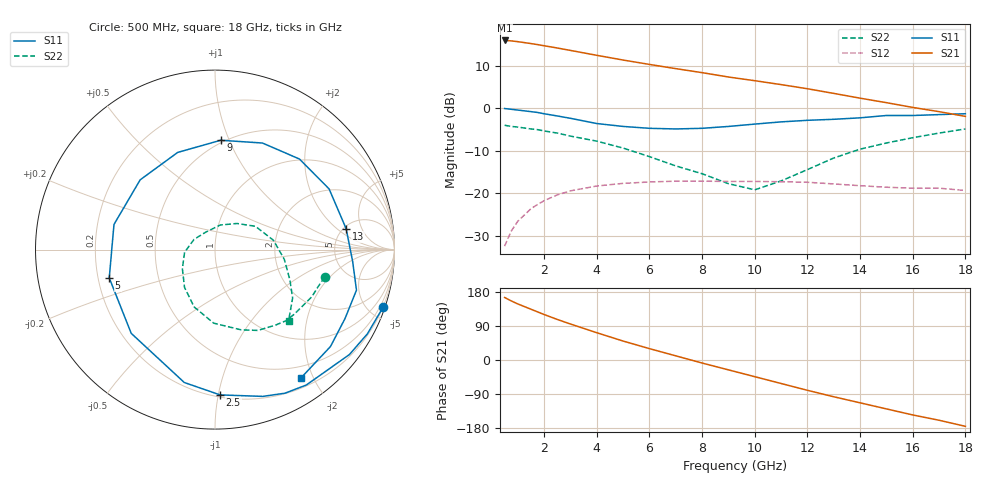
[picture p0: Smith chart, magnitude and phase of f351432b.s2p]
!ATF-35143
!S-PARAMETERS at Vds=2V  Id=10mA.  LAST UPDATED 06-3-99
# ghz s ma r 50
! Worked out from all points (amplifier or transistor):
!   23 points, 500 MHz to 18 GHz, reference 50 ohm
!   highest |S21| = 15.9 dB at 500 MHz (marker M1)
!   |S21| within 3 dB of that: start of sweep to 3.576 GHz
!   unconditionally stable (mu >= 1): 8.306 GHz to end of sweep
!   at 1.5 GHz: K = 0.23, MSG = 19.4 dB, |S12| = -23.6 dB
!   at 7 GHz: K = 0.88, MSG = 13.2 dB, |S12| = -17.1 dB
!   at 18 GHz: K = 1.41, MAG = 4.9 dB, |S12| = -19.3 dB
!   lowest NFmin = 0.10 dB at 500 MHz
!   S11 on the Smith chart (normalised r, x): 500 MHz: 0.18, -5.97; 2.5 GHz: 0.21, -1.01; 5 GHz: 0.25, -0.12; 9 GHz: 0.48, +0.93; 13 GHz: 5.27, +2.70; 18 GHz: 0.33, -1.83
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0.5  0.99 -19.0  6.23 165.0  0.024 78.0  0.63 -14.0
0.75  0.97 -29.0  6.16 156.0  0.036 71.0  0.61 -20.0
1  0.95 -38.0  6.03 148.0  0.047 65.0  0.6 -26.0
1.5  0.91 -56.0  5.73 134.0  0.066 54.0  0.57 -39.0
1.75  0.89 -64.0  5.57 127.0  0.074 49.0  0.56 -45.0
2  0.86 -72.0  5.4 120.0  0.082 44.0  0.54 -51.0
2.5  0.81 -88.0  5.08 107.0  0.096 35.0  0.51 -62.0
3  0.76 -103.0  4.76 95.0  0.107 26.0  0.47 -72.0
4  0.66 -135.0  4.17 72.0  0.122 9.0  0.41 -91.0
5  0.61 -165.0  3.67 50.0  0.131 -6.0  0.34 -110.0
6  0.58 166.0  3.26 30.0  0.136 -20.0  0.27 -129.0
7  0.57 137.0  2.91 11.0  0.139 -34.0  0.21 -150.0
8  0.58 111.0  2.61 -8.0  0.139 -46.0  0.17 -175.0
9  0.61 87.0  2.32 -26.0  0.138 -58.0  0.13 154.0
10  0.65 66.0  2.1 -44.0  0.138 -68.0  0.11 118.0
11  0.69 47.0  1.89 -62.0  0.137 -79.0  0.14 78.0
12  0.72 28.0  1.69 -80.0  0.135 -91.0  0.19 50.0
13  0.74 9.0  1.49 -97.0  0.129 -102.0  0.26 30.0
14  0.77 -5.0  1.31 -113.0  0.123 -111.0  0.33 9.0
15  0.82 -16.0  1.16 -129.0  0.118 -120.0  0.39 -8.0
16  0.82 -28.0  1.02 -145.0  0.115 -130.0  0.45 -22.0
18  0.86 -56.0  0.8 -175.0  0.108 -149.0  0.57 -44.0
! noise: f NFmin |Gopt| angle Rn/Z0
0.5  0.1  0.88  5  0.15
0.9  0.11  0.84  14  0.15
1.5  0.17  0.77  26  0.15
1.8  0.2  0.74  32  0.15
2.5  0.29  0.66  49  0.14
3  0.34  0.6  61  0.12
5  0.58  0.45  115  0.08
6  0.69  0.4  146  0.05
8  0.92  0.35  -149  0.07
10  1.16  0.37  -82  0.22
